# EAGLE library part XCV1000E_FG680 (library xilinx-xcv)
xcv1000e_fg680_1532 edit this description Auto generated by make-symbol-device-package-bsdl.ulp Rev. 26 Source: xcv1000e_fg680_1532.bsd
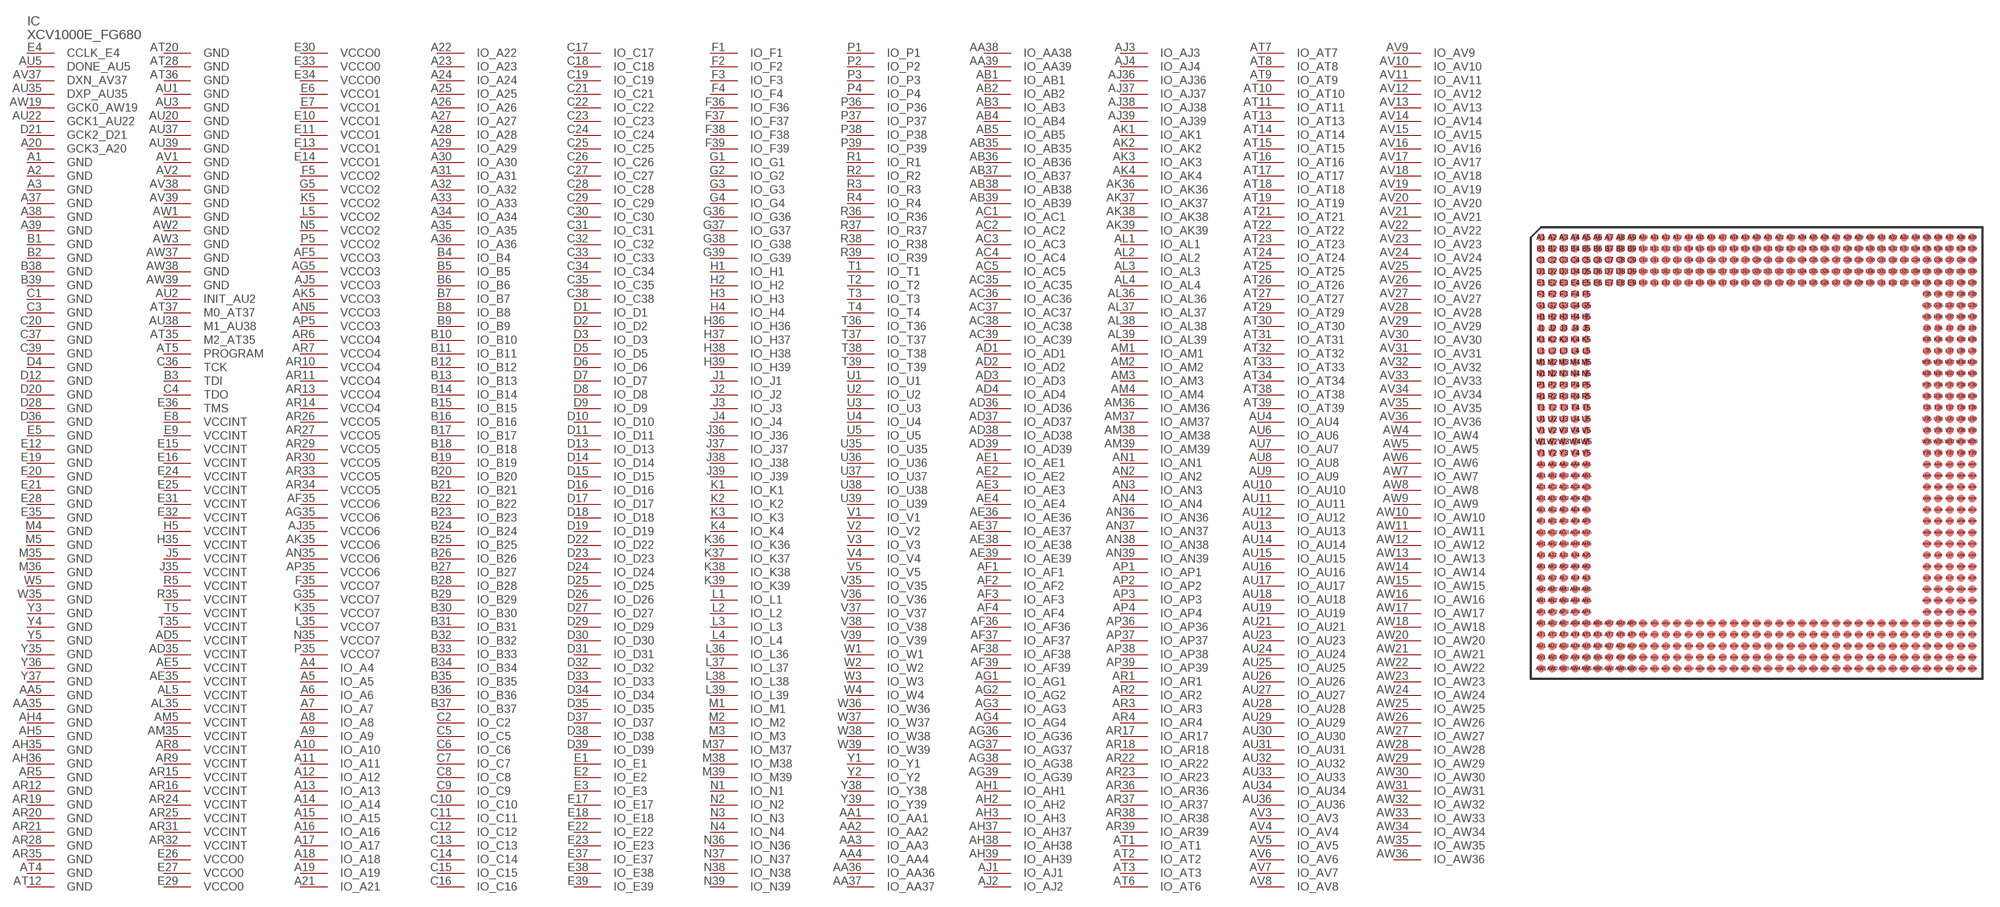
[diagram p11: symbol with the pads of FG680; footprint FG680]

Designator prefix IC

## XCV1000E_FG680 (OC_FARNELL: unknown; OC_NEWARK: unknown)  [FG680]
A1  GND  pwr
A2  GND  pwr
A3  GND  pwr
A4  IO_A4
A5  IO_A5
A6  IO_A6
A7  IO_A7
A8  IO_A8
A9  IO_A9
A10  IO_A10
A11  IO_A11
A12  IO_A12
A13  IO_A13
A14  IO_A14
A15  IO_A15
A16  IO_A16
A17  IO_A17
A18  IO_A18
A19  IO_A19
A20  GCK3_A20  in
A21  IO_A21
A22  IO_A22
A23  IO_A23
A24  IO_A24
A25  IO_A25
A26  IO_A26
A27  IO_A27
A28  IO_A28
A29  IO_A29
A30  IO_A30
A31  IO_A31
A32  IO_A32
A33  IO_A33
A34  IO_A34
A35  IO_A35
A36  IO_A36
A37  GND  pwr
A38  GND  pwr
A39  GND  pwr
AA1  IO_AA1
AA2  IO_AA2
AA3  IO_AA3
AA4  IO_AA4
AA5  GND  pwr
AA35  GND  pwr
AA36  IO_AA36
AA37  IO_AA37
AA38  IO_AA38
AA39  IO_AA39
AB1  IO_AB1
AB2  IO_AB2
AB3  IO_AB3
AB4  IO_AB4
AB5  IO_AB5
AB35  IO_AB35
AB36  IO_AB36
AB37  IO_AB37
AB38  IO_AB38
AB39  IO_AB39
AC1  IO_AC1
AC2  IO_AC2
AC3  IO_AC3
AC4  IO_AC4
AC5  IO_AC5
AC35  IO_AC35
AC36  IO_AC36
AC37  IO_AC37
AC38  IO_AC38
AC39  IO_AC39
AD1  IO_AD1
AD2  IO_AD2
AD3  IO_AD3
AD4  IO_AD4
AD5  VCCINT  pwr
AD35  VCCINT  pwr
AD36  IO_AD36
AD37  IO_AD37
AD38  IO_AD38
AD39  IO_AD39
AE1  IO_AE1
AE2  IO_AE2
AE3  IO_AE3
AE4  IO_AE4
AE5  VCCINT  pwr
AE35  VCCINT  pwr
AE36  IO_AE36
AE37  IO_AE37
AE38  IO_AE38
AE39  IO_AE39
AF1  IO_AF1
AF2  IO_AF2
AF3  IO_AF3
AF4  IO_AF4
AF5  VCCO3  pwr
AF35  VCCO6  pwr
AF36  IO_AF36
AF37  IO_AF37
AF38  IO_AF38
AF39  IO_AF39
AG1  IO_AG1
AG2  IO_AG2
AG3  IO_AG3
AG4  IO_AG4
AG5  VCCO3  pwr
AG35  VCCO6  pwr
AG36  IO_AG36
AG37  IO_AG37
AG38  IO_AG38
AG39  IO_AG39
AH1  IO_AH1
AH2  IO_AH2
AH3  IO_AH3
AH4  GND  pwr
AH5  GND  pwr
AH35  GND  pwr
AH36  GND  pwr
AH37  IO_AH37
AH38  IO_AH38
AH39  IO_AH39
AJ1  IO_AJ1
AJ2  IO_AJ2
AJ3  IO_AJ3
AJ4  IO_AJ4
AJ5  VCCO3  pwr
AJ35  VCCO6  pwr
AJ36  IO_AJ36
AJ37  IO_AJ37
AJ38  IO_AJ38
AJ39  IO_AJ39
AK1  IO_AK1
AK2  IO_AK2
AK3  IO_AK3
AK4  IO_AK4
AK5  VCCO3  pwr
AK35  VCCO6  pwr
AK36  IO_AK36
AK37  IO_AK37
AK38  IO_AK38
AK39  IO_AK39
AL1  IO_AL1
AL2  IO_AL2
AL3  IO_AL3
AL4  IO_AL4
AL5  VCCINT  pwr
AL35  VCCINT  pwr
AL36  IO_AL36
AL37  IO_AL37
AL38  IO_AL38
AL39  IO_AL39
AM1  IO_AM1
AM2  IO_AM2
AM3  IO_AM3
AM4  IO_AM4
AM5  VCCINT  pwr
AM35  VCCINT  pwr
AM36  IO_AM36
AM37  IO_AM37
AM38  IO_AM38
AM39  IO_AM39
AN1  IO_AN1
AN2  IO_AN2
AN3  IO_AN3
AN4  IO_AN4
AN5  VCCO3  pwr
AN35  VCCO6  pwr
AN36  IO_AN36
AN37  IO_AN37
AN38  IO_AN38
AN39  IO_AN39
AP1  IO_AP1
AP2  IO_AP2
AP3  IO_AP3
AP4  IO_AP4
AP5  VCCO3  pwr
AP35  VCCO6  pwr
AP36  IO_AP36
AP37  IO_AP37
AP38  IO_AP38
AP39  IO_AP39
AR1  IO_AR1
AR2  IO_AR2
AR3  IO_AR3
AR4  IO_AR4
AR5  GND  pwr
AR6  VCCO4  pwr
AR7  VCCO4  pwr
AR8  VCCINT  pwr
AR9  VCCINT  pwr
AR10  VCCO4  pwr
AR11  VCCO4  pwr
AR12  GND  pwr
AR13  VCCO4  pwr
AR14  VCCO4  pwr
AR15  VCCINT  pwr
AR16  VCCINT  pwr
AR17  IO_AR17
AR18  IO_AR18
AR19  GND  pwr
AR20  GND  pwr
AR21  GND  pwr
AR22  IO_AR22
AR23  IO_AR23
AR24  VCCINT  pwr
AR25  VCCINT  pwr
AR26  VCCO5  pwr
AR27  VCCO5  pwr
AR28  GND  pwr
AR29  VCCO5  pwr
AR30  VCCO5  pwr
AR31  VCCINT  pwr
AR32  VCCINT  pwr
AR33  VCCO5  pwr
AR34  VCCO5  pwr
AR35  GND  pwr
AR36  IO_AR36
AR37  IO_AR37
AR38  IO_AR38
AR39  IO_AR39
AT1  IO_AT1
AT2  IO_AT2
AT3  IO_AT3
AT4  GND  pwr
AT5  PROGRAM  in
AT6  IO_AT6
AT7  IO_AT7
AT8  IO_AT8
AT9  IO_AT9
AT10  IO_AT10
AT11  IO_AT11
AT12  GND  pwr
AT13  IO_AT13
AT14  IO_AT14
AT15  IO_AT15
AT16  IO_AT16
AT17  IO_AT17
AT18  IO_AT18
AT19  IO_AT19
AT20  GND  pwr
AT21  IO_AT21
AT22  IO_AT22
AT23  IO_AT23
AT24  IO_AT24
AT25  IO_AT25
AT26  IO_AT26
AT27  IO_AT27
AT28  GND  pwr
AT29  IO_AT29
AT30  IO_AT30
AT31  IO_AT31
AT32  IO_AT32
AT33  IO_AT33
AT34  IO_AT34
AT35  M2_AT35  in
AT36  GND  pwr
AT37  M0_AT37  in
AT38  IO_AT38
AT39  IO_AT39
AU1  GND  pwr
AU2  INIT_AU2
AU3  GND  pwr
AU4  IO_AU4
AU5  DONE_AU5
AU6  IO_AU6
AU7  IO_AU7
AU8  IO_AU8
AU9  IO_AU9
AU10  IO_AU10
AU11  IO_AU11
AU12  IO_AU12
AU13  IO_AU13
AU14  IO_AU14
AU15  IO_AU15
AU16  IO_AU16
AU17  IO_AU17
AU18  IO_AU18
AU19  IO_AU19
AU20  GND  pwr
AU21  IO_AU21
AU22  GCK1_AU22  in
AU23  IO_AU23
AU24  IO_AU24
AU25  IO_AU25
AU26  IO_AU26
AU27  IO_AU27
AU28  IO_AU28
AU29  IO_AU29
AU30  IO_AU30
AU31  IO_AU31
AU32  IO_AU32
AU33  IO_AU33
AU34  IO_AU34
AU35  DXP_AU35  pas
AU36  IO_AU36
AU37  GND  pwr
AU38  M1_AU38  in
AU39  GND  pwr
AV1  GND  pwr
AV2  GND  pwr
AV3  IO_AV3
AV4  IO_AV4
AV5  IO_AV5
AV6  IO_AV6
AV7  IO_AV7
AV8  IO_AV8
AV9  IO_AV9
AV10  IO_AV10
AV11  IO_AV11
AV12  IO_AV12
AV13  IO_AV13
AV14  IO_AV14
AV15  IO_AV15
AV16  IO_AV16
AV17  IO_AV17
AV18  IO_AV18
AV19  IO_AV19
AV20  IO_AV20
AV21  IO_AV21
AV22  IO_AV22
AV23  IO_AV23
AV24  IO_AV24
AV25  IO_AV25
AV26  IO_AV26
AV27  IO_AV27
AV28  IO_AV28
AV29  IO_AV29
AV30  IO_AV30
AV31  IO_AV31
AV32  IO_AV32
AV33  IO_AV33
AV34  IO_AV34
AV35  IO_AV35
AV36  IO_AV36
AV37  DXN_AV37  pas
AV38  GND  pwr
AV39  GND  pwr
AW1  GND  pwr
AW2  GND  pwr
AW3  GND  pwr
AW4  IO_AW4
AW5  IO_AW5
AW6  IO_AW6
AW7  IO_AW7
AW8  IO_AW8
AW9  IO_AW9
AW10  IO_AW10
AW11  IO_AW11
AW12  IO_AW12
AW13  IO_AW13
AW14  IO_AW14
AW15  IO_AW15
AW16  IO_AW16
AW17  IO_AW17
AW18  IO_AW18
AW19  GCK0_AW19  in
AW20  IO_AW20
AW21  IO_AW21
AW22  IO_AW22
AW23  IO_AW23
AW24  IO_AW24
AW25  IO_AW25
AW26  IO_AW26
AW27  IO_AW27
AW28  IO_AW28
AW29  IO_AW29
AW30  IO_AW30
AW31  IO_AW31
AW32  IO_AW32
AW33  IO_AW33
AW34  IO_AW34
AW35  IO_AW35
AW36  IO_AW36
AW37  GND  pwr
AW38  GND  pwr
AW39  GND  pwr
B1  GND  pwr
B2  GND  pwr
B3  TDI  in
B4  IO_B4
B5  IO_B5
B6  IO_B6
B7  IO_B7
B8  IO_B8
B9  IO_B9
B10  IO_B10
B11  IO_B11
B12  IO_B12
B13  IO_B13
B14  IO_B14
B15  IO_B15
B16  IO_B16
B17  IO_B17
B18  IO_B18
B19  IO_B19
B20  IO_B20
B21  IO_B21
B22  IO_B22
B23  IO_B23
B24  IO_B24
B25  IO_B25
B26  IO_B26
B27  IO_B27
B28  IO_B28
B29  IO_B29
B30  IO_B30
B31  IO_B31
B32  IO_B32
B33  IO_B33
B34  IO_B34
B35  IO_B35
B36  IO_B36
B37  IO_B37
B38  GND  pwr
B39  GND  pwr
C1  GND  pwr
C2  IO_C2
C3  GND  pwr
C4  TDO  out
C5  IO_C5
C6  IO_C6
C7  IO_C7
C8  IO_C8
C9  IO_C9
C10  IO_C10
C11  IO_C11
C12  IO_C12
C13  IO_C13
C14  IO_C14
C15  IO_C15
C16  IO_C16
C17  IO_C17
C18  IO_C18
C19  IO_C19
C20  GND  pwr
C21  IO_C21
C22  IO_C22
C23  IO_C23
C24  IO_C24
C25  IO_C25
C26  IO_C26
C27  IO_C27
C28  IO_C28
C29  IO_C29
C30  IO_C30
C31  IO_C31
C32  IO_C32
C33  IO_C33
C34  IO_C34
C35  IO_C35
C36  TCK  in
C37  GND  pwr
C38  IO_C38
C39  GND  pwr
D1  IO_D1
D2  IO_D2
D3  IO_D3
D4  GND  pwr
D5  IO_D5
D6  IO_D6
D7  IO_D7
D8  IO_D8
D9  IO_D9
D10  IO_D10
D11  IO_D11
D12  GND  pwr
D13  IO_D13
D14  IO_D14
D15  IO_D15
D16  IO_D16
D17  IO_D17
D18  IO_D18
D19  IO_D19
D20  GND  pwr
D21  GCK2_D21  in
D22  IO_D22
D23  IO_D23
D24  IO_D24
D25  IO_D25
D26  IO_D26
D27  IO_D27
D28  GND  pwr
D29  IO_D29
D30  IO_D30
D31  IO_D31
D32  IO_D32
D33  IO_D33
D34  IO_D34
D35  IO_D35
D36  GND  pwr
D37  IO_D37
D38  IO_D38
D39  IO_D39
E1  IO_E1
E2  IO_E2
E3  IO_E3
E4  CCLK_E4
E5  GND  pwr
E6  VCCO1  pwr
E7  VCCO1  pwr
E8  VCCINT  pwr
E9  VCCINT  pwr
E10  VCCO1  pwr
E11  VCCO1  pwr
E12  GND  pwr
E13  VCCO1  pwr
E14  VCCO1  pwr
E15  VCCINT  pwr
E16  VCCINT  pwr
E17  IO_E17
E18  IO_E18
E19  GND  pwr
E20  GND  pwr
E21  GND  pwr
E22  IO_E22
E23  IO_E23
E24  VCCINT  pwr
E25  VCCINT  pwr
E26  VCCO0  pwr
E27  VCCO0  pwr
E28  GND  pwr
E29  VCCO0  pwr
E30  VCCO0  pwr
E31  VCCINT  pwr
E32  VCCINT  pwr
E33  VCCO0  pwr
E34  VCCO0  pwr
E35  GND  pwr
E36  TMS  in
E37  IO_E37
E38  IO_E38
E39  IO_E39
F1  IO_F1
F2  IO_F2
F3  IO_F3
F4  IO_F4
F5  VCCO2  pwr
F35  VCCO7  pwr
F36  IO_F36
F37  IO_F37
F38  IO_F38
F39  IO_F39
G1  IO_G1
G2  IO_G2
G3  IO_G3
G4  IO_G4
G5  VCCO2  pwr
G35  VCCO7  pwr
G36  IO_G36
G37  IO_G37
G38  IO_G38
G39  IO_G39
H1  IO_H1
H2  IO_H2
H3  IO_H3
H4  IO_H4
H5  VCCINT  pwr
H35  VCCINT  pwr
H36  IO_H36
H37  IO_H37
H38  IO_H38
H39  IO_H39
J1  IO_J1
J2  IO_J2
J3  IO_J3
J4  IO_J4
J5  VCCINT  pwr
J35  VCCINT  pwr
J36  IO_J36
J37  IO_J37
J38  IO_J38
J39  IO_J39
K1  IO_K1
K2  IO_K2
K3  IO_K3
K4  IO_K4
K5  VCCO2  pwr
K35  VCCO7  pwr
K36  IO_K36
K37  IO_K37
K38  IO_K38
K39  IO_K39
L1  IO_L1
L2  IO_L2
L3  IO_L3
L4  IO_L4
L5  VCCO2  pwr
L35  VCCO7  pwr
L36  IO_L36
L37  IO_L37
L38  IO_L38
L39  IO_L39
M1  IO_M1
M2  IO_M2
M3  IO_M3
M4  GND  pwr
M5  GND  pwr
M35  GND  pwr
M36  GND  pwr
M37  IO_M37
M38  IO_M38
M39  IO_M39
N1  IO_N1
N2  IO_N2
N3  IO_N3
N4  IO_N4
N5  VCCO2  pwr
N35  VCCO7  pwr
N36  IO_N36
N37  IO_N37
N38  IO_N38
N39  IO_N39
P1  IO_P1
P2  IO_P2
P3  IO_P3
P4  IO_P4
P5  VCCO2  pwr
P35  VCCO7  pwr
P36  IO_P36
P37  IO_P37
P38  IO_P38
P39  IO_P39
R1  IO_R1
R2  IO_R2
R3  IO_R3
R4  IO_R4
R5  VCCINT  pwr
R35  VCCINT  pwr
R36  IO_R36
R37  IO_R37
R38  IO_R38
R39  IO_R39
T1  IO_T1
T2  IO_T2
T3  IO_T3
T4  IO_T4
T5  VCCINT  pwr
T35  VCCINT  pwr
T36  IO_T36
T37  IO_T37
T38  IO_T38
T39  IO_T39
U1  IO_U1
U2  IO_U2
U3  IO_U3
U4  IO_U4
U5  IO_U5
U35  IO_U35
U36  IO_U36
U37  IO_U37
U38  IO_U38
U39  IO_U39
V1  IO_V1
V2  IO_V2
V3  IO_V3
V4  IO_V4
V5  IO_V5
V35  IO_V35
V36  IO_V36
V37  IO_V37
V38  IO_V38
V39  IO_V39
W1  IO_W1
W2  IO_W2
W3  IO_W3
W4  IO_W4
W5  GND  pwr
W35  GND  pwr
W36  IO_W36
W37  IO_W37
W38  IO_W38
W39  IO_W39
Y1  IO_Y1
Y2  IO_Y2
Y3  GND  pwr
Y4  GND  pwr
Y5  GND  pwr
Y35  GND  pwr
Y36  GND  pwr
Y37  GND  pwr
Y38  IO_Y38
Y39  IO_Y39

## Footprint FG680 (pad centres in mm)
xcv1000_fg680_1532 edit this description Auto generated by make-symbol-device-package-bsdl.ulp Rev. 26 Source: xcv1000_fg680_1532.bsd
smd 0.7 x 0.7: A1 -19,19; A2 -18,19; A3 -17,19; A4 -16,19; A5 -15,19; A6 -14,19; A7 -13,19; A8 -12,19; A9 -11,19; A10 -10,19; A11 -9,19; A12 -8,19; A13 -7,19; A14 -6,19; A15 -5,19; A16 -4,19; A17 -3,19; A18 -2,19; A19 -1,19; A20 0,19; A21 1,19; A22 2,19; A23 3,19; A24 4,19; A25 5,19; A26 6,19; A27 7,19; A28 8,19; A29 9,19; A30 10,19; A31 11,19; A32 12,19; A33 13,19; A34 14,19; A35 15,19; A36 16,19; A37 17,19; A38 18,19; A39 19,19; AA1 -19,-1; AA2 -18,-1; AA3 -17,-1; AA4 -16,-1; AA5 -15,-1; AA35 15,-1; AA36 16,-1; AA37 17,-1; AA38 18,-1; AA39 19,-1; AB1 -19,-2; AB2 -18,-2; AB3 -17,-2; AB4 -16,-2; AB5 -15,-2; AB35 15,-2; AB36 16,-2; AB37 17,-2; AB38 18,-2; AB39 19,-2; AC1 -19,-3; AC2 -18,-3; AC3 -17,-3; AC4 -16,-3; AC5 -15,-3; AC35 15,-3; AC36 16,-3; AC37 17,-3; AC38 18,-3; AC39 19,-3; AD1 -19,-4; AD2 -18,-4; AD3 -17,-4; AD4 -16,-4; AD5 -15,-4; AD35 15,-4; AD36 16,-4; AD37 17,-4; AD38 18,-4; AD39 19,-4; AE1 -19,-5; AE2 -18,-5; AE3 -17,-5; AE4 -16,-5; AE5 -15,-5; AE35 15,-5; AE36 16,-5; AE37 17,-5; AE38 18,-5; AE39 19,-5; AF1 -19,-6; AF2 -18,-6; AF3 -17,-6; AF4 -16,-6; AF5 -15,-6; AF35 15,-6; AF36 16,-6; AF37 17,-6; AF38 18,-6; AF39 19,-6; AG1 -19,-7; AG2 -18,-7; AG3 -17,-7; AG4 -16,-7; AG5 -15,-7; AG35 15,-7; AG36 16,-7; AG37 17,-7; AG38 18,-7; AG39 19,-7; AH1 -19,-8; AH2 -18,-8; AH3 -17,-8; AH4 -16,-8; AH5 -15,-8; AH35 15,-8; AH36 16,-8; AH37 17,-8; AH38 18,-8; AH39 19,-8; AJ1 -19,-9; AJ2 -18,-9; AJ3 -17,-9; AJ4 -16,-9; AJ5 -15,-9; AJ35 15,-9; AJ36 16,-9; AJ37 17,-9; AJ38 18,-9; AJ39 19,-9; AK1 -19,-10; AK2 -18,-10; AK3 -17,-10; AK4 -16,-10; AK5 -15,-10; AK35 15,-10; AK36 16,-10; AK37 17,-10; AK38 18,-10; AK39 19,-10; AL1 -19,-11; AL2 -18,-11; AL3 -17,-11; AL4 -16,-11; AL5 -15,-11; AL35 15,-11; AL36 16,-11; AL37 17,-11; AL38 18,-11; AL39 19,-11; AM1 -19,-12; AM2 -18,-12; AM3 -17,-12; AM4 -16,-12; AM5 -15,-12; AM35 15,-12; AM36 16,-12; AM37 17,-12; AM38 18,-12; AM39 19,-12; AN1 -19,-13; AN2 -18,-13; AN3 -17,-13; AN4 -16,-13; AN5 -15,-13; AN35 15,-13; AN36 16,-13; AN37 17,-13; AN38 18,-13; AN39 19,-13; AP1 -19,-14; AP2 -18,-14; AP3 -17,-14; AP4 -16,-14; AP5 -15,-14; AP35 15,-14; AP36 16,-14; AP37 17,-14; AP38 18,-14; AP39 19,-14; AR1 -19,-15; AR2 -18,-15; AR3 -17,-15; AR4 -16,-15; AR5 -15,-15; AR6 -14,-15; AR7 -13,-15; AR8 -12,-15; AR9 -11,-15; AR10 -10,-15; AR11 -9,-15; AR12 -8,-15; AR13 -7,-15; AR14 -6,-15; AR15 -5,-15; AR16 -4,-15; AR17 -3,-15; AR18 -2,-15; AR19 -1,-15; AR20 0,-15; AR21 1,-15; AR22 2,-15; AR23 3,-15; AR24 4,-15; AR25 5,-15; AR26 6,-15; AR27 7,-15; AR28 8,-15; AR29 9,-15; AR30 10,-15; AR31 11,-15; AR32 12,-15; AR33 13,-15; AR34 14,-15; AR35 15,-15; AR36 16,-15; AR37 17,-15; AR38 18,-15; AR39 19,-15; AT1 -19,-16; AT2 -18,-16; AT3 -17,-16; AT4 -16,-16; AT5 -15,-16; AT6 -14,-16; AT7 -13,-16; AT8 -12,-16; AT9 -11,-16; AT10 -10,-16; AT11 -9,-16; AT12 -8,-16; AT13 -7,-16; AT14 -6,-16; AT15 -5,-16; AT16 -4,-16; AT17 -3,-16; AT18 -2,-16; AT19 -1,-16; AT20 0,-16; AT21 1,-16; AT22 2,-16; AT23 3,-16; AT24 4,-16; AT25 5,-16; AT26 6,-16; AT27 7,-16; AT28 8,-16; AT29 9,-16; AT30 10,-16; AT31 11,-16; AT32 12,-16; AT33 13,-16; AT34 14,-16; AT35 15,-16; AT36 16,-16; AT37 17,-16; AT38 18,-16; AT39 19,-16; AU1 -19,-17; AU2 -18,-17; AU3 -17,-17; AU4 -16,-17; AU5 -15,-17; AU6 -14,-17; AU7 -13,-17; AU8 -12,-17; AU9 -11,-17; AU10 -10,-17; AU11 -9,-17; AU12 -8,-17; AU13 -7,-17; AU14 -6,-17; AU15 -5,-17; AU16 -4,-17; AU17 -3,-17; AU18 -2,-17; AU19 -1,-17; AU20 0,-17; AU21 1,-17; AU22 2,-17; AU23 3,-17; AU24 4,-17; AU25 5,-17; AU26 6,-17; AU27 7,-17; AU28 8,-17; AU29 9,-17; AU30 10,-17; AU31 11,-17; AU32 12,-17; AU33 13,-17; AU34 14,-17; AU35 15,-17; AU36 16,-17; AU37 17,-17; AU38 18,-17; AU39 19,-17; AV1 -19,-18; AV2 -18,-18; AV3 -17,-18; AV4 -16,-18; AV5 -15,-18; AV6 -14,-18; AV7 -13,-18; AV8 -12,-18; AV9 -11,-18; AV10 -10,-18; AV11 -9,-18; AV12 -8,-18; AV13 -7,-18; AV14 -6,-18; AV15 -5,-18; AV16 -4,-18; AV17 -3,-18; AV18 -2,-18; AV19 -1,-18; AV20 0,-18; AV21 1,-18; AV22 2,-18; AV23 3,-18; AV24 4,-18; AV25 5,-18; AV26 6,-18; AV27 7,-18; AV28 8,-18; AV29 9,-18; AV30 10,-18; AV31 11,-18; AV32 12,-18; AV33 13,-18; AV34 14,-18; AV35 15,-18; AV36 16,-18; AV37 17,-18; AV38 18,-18; AV39 19,-18; AW1 -19,-19; AW2 -18,-19; AW3 -17,-19; AW4 -16,-19; AW5 -15,-19; AW6 -14,-19; AW7 -13,-19; AW8 -12,-19; AW9 -11,-19; AW10 -10,-19; AW11 -9,-19; AW12 -8,-19; AW13 -7,-19; AW14 -6,-19; AW15 -5,-19; AW16 -4,-19; AW17 -3,-19; AW18 -2,-19; AW19 -1,-19; AW20 0,-19; AW21 1,-19; AW22 2,-19; AW23 3,-19; AW24 4,-19; AW25 5,-19; AW26 6,-19; AW27 7,-19; AW28 8,-19; AW29 9,-19; AW30 10,-19; AW31 11,-19; AW32 12,-19; AW33 13,-19; AW34 14,-19; AW35 15,-19; AW36 16,-19; AW37 17,-19; AW38 18,-19; AW39 19,-19; B1 -19,18; B2 -18,18; B3 -17,18; B4 -16,18; B5 -15,18; B6 -14,18; B7 -13,18; B8 -12,18; B9 -11,18; B10 -10,18; B11 -9,18; B12 -8,18; B13 -7,18; B14 -6,18; B15 -5,18; B16 -4,18; B17 -3,18; B18 -2,18; B19 -1,18; B20 0,18; B21 1,18; B22 2,18; B23 3,18; B24 4,18; B25 5,18; B26 6,18; B27 7,18; B28 8,18; B29 9,18; B30 10,18; B31 11,18; B32 12,18; B33 13,18; B34 14,18; B35 15,18; B36 16,18; B37 17,18; B38 18,18; B39 19,18; C1 -19,17; C2 -18,17; C3 -17,17; C4 -16,17; C5 -15,17; C6 -14,17; C7 -13,17; C8 -12,17; C9 -11,17; C10 -10,17; C11 -9,17; C12 -8,17; C13 -7,17; C14 -6,17; C15 -5,17; C16 -4,17; C17 -3,17; C18 -2,17; C19 -1,17; C20 0,17; C21 1,17; C22 2,17; C23 3,17; C24 4,17; C25 5,17; C26 6,17; C27 7,17; C28 8,17; C29 9,17; C30 10,17; C31 11,17; C32 12,17; C33 13,17; C34 14,17; C35 15,17; C36 16,17; C37 17,17; C38 18,17; C39 19,17; D1 -19,16; D2 -18,16; D3 -17,16; D4 -16,16; D5 -15,16; D6 -14,16; D7 -13,16; D8 -12,16; D9 -11,16; D10 -10,16; D11 -9,16; D12 -8,16; D13 -7,16; D14 -6,16; D15 -5,16; D16 -4,16; D17 -3,16; D18 -2,16; D19 -1,16; D20 0,16; D21 1,16; D22 2,16; D23 3,16; D24 4,16; D25 5,16; D26 6,16; D27 7,16; D28 8,16; D29 9,16; D30 10,16; D31 11,16; D32 12,16; D33 13,16; D34 14,16; D35 15,16; D36 16,16; D37 17,16; D38 18,16; D39 19,16; E1 -19,15; E2 -18,15; E3 -17,15; E4 -16,15; E5 -15,15; E6 -14,15; E7 -13,15; E8 -12,15; E9 -11,15; E10 -10,15; E11 -9,15; E12 -8,15; E13 -7,15; E14 -6,15; E15 -5,15; E16 -4,15; E17 -3,15; E18 -2,15; E19 -1,15; E20 0,15; E21 1,15; E22 2,15; E23 3,15; E24 4,15; E25 5,15; E26 6,15; E27 7,15; E28 8,15; E29 9,15; E30 10,15; E31 11,15; E32 12,15; E33 13,15; E34 14,15; E35 15,15; E36 16,15; E37 17,15; E38 18,15; E39 19,15; F1 -19,14; F2 -18,14; F3 -17,14; F4 -16,14; F5 -15,14; F35 15,14; F36 16,14; F37 17,14; F38 18,14; F39 19,14; G1 -19,13; G2 -18,13; G3 -17,13; G4 -16,13; G5 -15,13; G35 15,13; G36 16,13; G37 17,13; G38 18,13; G39 19,13; H1 -19,12; H2 -18,12; H3 -17,12; H4 -16,12; H5 -15,12; H35 15,12; H36 16,12; H37 17,12; H38 18,12; H39 19,12; J1 -19,11; J2 -18,11; J3 -17,11; J4 -16,11; J5 -15,11; J35 15,11; J36 16,11; J37 17,11; J38 18,11; J39 19,11; K1 -19,10; K2 -18,10; K3 -17,10; K4 -16,10; K5 -15,10; K35 15,10; K36 16,10; K37 17,10; K38 18,10; K39 19,10; L1 -19,9; L2 -18,9; L3 -17,9; L4 -16,9; L5 -15,9; L35 15,9; L36 16,9; L37 17,9; L38 18,9; L39 19,9; M1 -19,8; M2 -18,8; M3 -17,8; M4 -16,8; M5 -15,8; M35 15,8; M36 16,8; M37 17,8; M38 18,8; M39 19,8; N1 -19,7; N2 -18,7; N3 -17,7; N4 -16,7; N5 -15,7; N35 15,7; N36 16,7; N37 17,7; N38 18,7; N39 19,7; P1 -19,6; P2 -18,6; P3 -17,6; P4 -16,6; P5 -15,6; P35 15,6; P36 16,6; P37 17,6; P38 18,6; P39 19,6; R1 -19,5; R2 -18,5; R3 -17,5; R4 -16,5; R5 -15,5; R35 15,5; R36 16,5; R37 17,5; R38 18,5; R39 19,5; T1 -19,4; T2 -18,4; T3 -17,4; T4 -16,4; T5 -15,4; T35 15,4; T36 16,4; T37 17,4; T38 18,4; T39 19,4; U1 -19,3; U2 -18,3; U3 -17,3; U4 -16,3; U5 -15,3; U35 15,3; U36 16,3; U37 17,3; U38 18,3; U39 19,3; V1 -19,2; V2 -18,2; V3 -17,2; V4 -16,2; V5 -15,2; V35 15,2; V36 16,2; V37 17,2; V38 18,2; V39 19,2; W1 -19,1; W2 -18,1; W3 -17,1; W4 -16,1; W5 -15,1; W35 15,1; W36 16,1; W37 17,1; W38 18,1; W39 19,1; Y1 -19,0; Y2 -18,0; Y3 -17,0; Y4 -16,0; Y5 -15,0; Y35 15,0; Y36 16,0; Y37 17,0; Y38 18,0; Y39 19,0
